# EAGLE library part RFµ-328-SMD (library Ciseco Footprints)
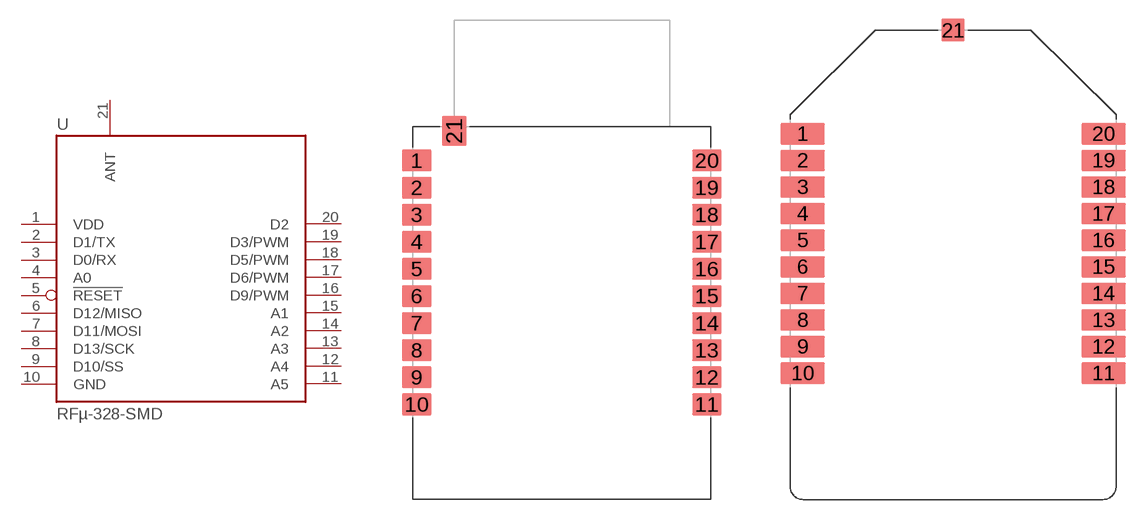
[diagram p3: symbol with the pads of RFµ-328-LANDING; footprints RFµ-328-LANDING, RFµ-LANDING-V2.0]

Designator prefix U

## RFµ-328-SMD  [RFµ-328-LANDING]
1  VDD  pwr
2  D1/TX  out
3  D0/RX  in
4  A0
5  !RESET  in
6  D12/MISO
7  D11/MOSI
8  D13/SCK
9  D10/SS
10  GND  pwr
11  A5
12  A4  out
13  A3
14  A2
15  A1
16  D9/PWM  in
17  D6/PWM
18  D5/PWM
19  D3/PWM
20  D2
21  ANT  out

## RFµ-328-SMD-V2.0  [RFµ-LANDING-V2.0]
Pads as for RFµ-328-LANDING

## Footprint RFµ-328-LANDING (pad centres in mm)
smd 2.2 x 1.6: 1 -10.7,20; 2 -10.7,18; 3 -10.7,16; 4 -10.7,14; 5 -10.7,12; 6 -10.7,10; 7 -10.7,8; 8 -10.7,6; 9 -10.7,4; 10 -10.7,2; 11 10.7,2; 12 10.7,4; 13 10.7,6; 14 10.7,8; 15 10.7,10; 16 10.7,12; 17 10.7,14; 18 10.7,16; 19 10.7,18; 20 10.7,20
smd 1.8 x 2.2: 21 -7.93,22.2

## Footprint RFµ-LANDING-V2.0 (pad centres in mm)
smd 3.35 x 1.6: 1 -11.3,20; 2 -11.3,18; 3 -11.3,16; 4 -11.3,14; 5 -11.3,12; 6 -11.3,10; 7 -11.3,8; 8 -11.3,6; 9 -11.3,4; 10 -11.3,2; 11 11.3,2; 12 11.3,4; 13 11.3,6; 14 11.3,8; 15 11.3,10; 16 11.3,12; 17 11.3,14; 18 11.3,16; 19 11.3,18; 20 11.3,20
smd 1.7 x 1.7: 21 0,27.8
